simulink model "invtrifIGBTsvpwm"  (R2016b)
settings: Solver=VariableStepAuto  StartTime=0.0  StopTime=5  RelTol=1e-3
libraries: powerlib x17, powerlib_meascontrol x4

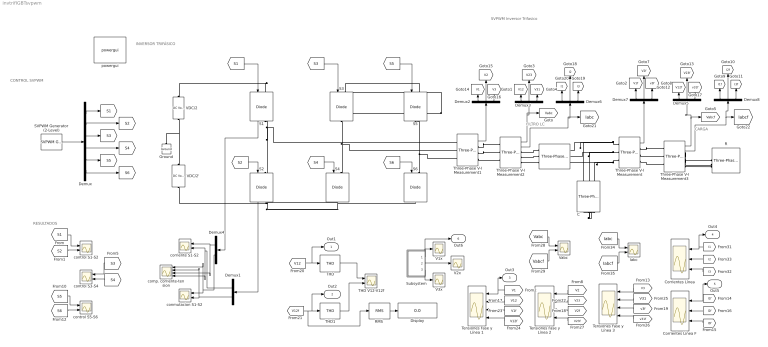
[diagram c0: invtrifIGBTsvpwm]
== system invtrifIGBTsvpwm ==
  note: RESULTADOS
  note: CONTROL SVPWM
  note: INVERSOR TRIFÁSICO
  note: SVPWM Inversor Trifasico
  note: CARGA
  note: FILTRO LC
  "C  " : powerlib/Elements/Three-Phase Series RLC Branch  LConnTagsString=A|B|C  RConnTagsString=A|B|C  BranchType=C  Resistance=1  Inductance=1e-3  Capacitance=1e-4  Measurements=None
  Corrientes Línea : Scope  NumInputPorts=3
  Corrientes Línea F : Scope  NumInputPorts=3
  Demux : Demux  Outputs=6
  Demux1 : Demux  Outputs=2
  Demux{2..3,5..8} (6 alike) : Demux  Outputs=3
  Demux4 : Demux  Outputs=2
  Display : Display
  Ground : powerlib/Elements/Ground  LConnTagsString=a
  Iabc : Scope  NumInputPorts=2
  L : powerlib/Elements/Three-Phase Series RLC Branch  LConnTagsString=A|B|C  RConnTagsString=A|B|C  BranchType=L  Resistance=40  Inductance=10e-3  Capacitance=1e-6  Measurements=Branch voltages and currents
  R : powerlib/Elements/Three-Phase Series RLC Load  LConnTagsString=A|B|C  Configuration=Y (grounded)  NominalVoltage=220  Vabc=[1e3 1e3 1e3]  Vabcp=[1e3 1e3 1e3]  NominalFrequency=50  UnbalancedPower=off  ActivePower=2430  InductivePower=1177  CapacitivePower=0  Pabc=[10e3 9e3 11e3]  QLabc=[100 90 110]  QCabc=[100 90 110]  Pabcp=[10e3 9e3 11e3]  QLabcp=[100 90 110]  QCabcp=[100 90 110]  Measurements=None  LoadType=constant Z
  "RMS " : powerlib_meascontrol/Measurements/RMS  TrueRMS=on  Freq=60  RMSInit=220  Ts=0
  S1 : powerlib/Power Electronics/IGBT//Diode  Ron=1e-3  Rs=1e5  Cs=inf  Measurements=on
  S2 : powerlib/Power Electronics/IGBT//Diode  Ron=1e-3  Rs=1e5  Cs=inf  Measurements=on
  S{3..6} (4 alike) : powerlib/Power Electronics/IGBT//Diode  Ron=1e-3  Rs=1e5  Cs=inf  Measurements=off
  SVPWM Generator (2-Level) : powerlib_meascontrol/Pulse & Signal Generators/SVPWM Generator (2-Level)  InputType=Internally generated  SwitchingPattern=Pattern #1  Fc=1050  ParUref=[0.85 -14 50]  Ts=0
  Subsystem : Subsystem
  THD : powerlib_meascontrol/Measurements/THD  Freq=60  Ts=0
  THD V12-V12f : Scope  NumInputPorts=2
  THD1 : powerlib_meascontrol/Measurements/THD  Freq=60  Ts=0
  Tensiones Fase y Línea 1 : Scope  NumInputPorts=4
  Tensiones Fase y Línea 2 : Scope  NumInputPorts=4
  Tensiones Fase y Línea 3 : Scope  NumInputPorts=4
  Three-Phase V-I Measurement : powerlib/Measurements/Three-Phase V-I Measurement  VoltageMeasurement=phase-to-ground  SetLabelV=off  LabelV=Vabc  Vpu=off  VpuLL=off  CurrentMeasurement=no  SetLabelI=off  LabelI=Iabc  Ipu=off  Pbase=100e6  Vbase=500e3  OutputType=Complex  PhasorSimulation=off  PSBequivalent=0
  Three-Phase V-I Measurement1 : powerlib/Measurements/Three-Phase V-I Measurement  VoltageMeasurement=phase-to-ground  SetLabelV=off  LabelV=Vabc  Vpu=off  VpuLL=off  CurrentMeasurement=no  SetLabelI=off  LabelI=Iabc  Ipu=off  Pbase=100e6  Vbase=500e3  OutputType=Complex  PhasorSimulation=off  PSBequivalent=0
  Three-Phase V-I Measurement2 : powerlib/Measurements/Three-Phase V-I Measurement  VoltageMeasurement=phase-to-phase  SetLabelV=off  LabelV=Vabc  Vpu=off  VpuLL=off  CurrentMeasurement=yes  SetLabelI=off  LabelI=Iabc  Ipu=off  Pbase=100e6  Vbase=500e3  OutputType=Complex  PhasorSimulation=off  PSBequivalent=0
  Three-Phase V-I Measurement3 : powerlib/Measurements/Three-Phase V-I Measurement  VoltageMeasurement=phase-to-phase  SetLabelV=off  LabelV=Vabc  Vpu=off  VpuLL=off  CurrentMeasurement=yes  SetLabelI=off  LabelI=Iabc  Ipu=off  Pbase=100e6  Vbase=500e3  OutputType=Complex  PhasorSimulation=off  PSBequivalent=0
  V1x : Scope
  V2x : Scope
  V3x : Scope
  VDC/2 : powerlib/Electrical Sources/DC Voltage Source  Amplitude=185  Measurements=None
  VDC/2' : powerlib/Electrical Sources/DC Voltage Source  Amplitude=185  Measurements=None
  "Vabc " : Scope  NumInputPorts=2
  comp. corriente-tension : Scope  NumInputPorts=4
  conmutacion S1-S2 : Scope  NumInputPorts=2
  control S1-S2 : Scope  NumInputPorts=2
  control S3-S4 : Scope  NumInputPorts=2
  "control S5-S6 " : Scope  NumInputPorts=2
  corriente S1-S2 : Scope  NumInputPorts=2
  powergui : powerlib/powergui  Priority=1  SimulationMode=Continuous  SolverType=Tustin/Backward Euler (TBE)  SampleTime=5e-5  frequency=60  SPID=off  DisableSnubberDevices=off  DisableRonSwitches=off  DisableVfSwitches=off  SwTol=0  DisplayEquations=off  Interpol=off  ExternalGateDelay=off  methode=off  Ts=10  FunctionMessages=off  echomessages=off  HookPort=off  EnableUseOfTLC=off  x0status=blocks  frequencyindice=0  Pbase=100e6  ErrMax=1e-4  Iterations=50  UnitsV=kV  UnitsW=MW  buscounter=0  RestoreLinks=warning  ResistiveCurrentMeasurement=off  Frange=[0:2:500]  Ylog=off  Xlog=on  ShowGrid=off  save=off  variable=ZData  structure=yout  ZoomFFT=off  StartTime=0.055  cycles=1  DisplayStyle=4  fundamental=50  FreqAxis=off  MaxFrequency=7800  frequencyindicesteady=1  RmsSteady=1  display=off
  Out1 : Outport  SignalName=V12
  Out2 : Outport  Port=2  SignalName=V12f
  Out3 : Outport  Port=3  SignalName=V1
  Out4 : Outport  Port=4  SignalName=I1
  Out5 : Outport  Port=5  SignalName=I1f
  Out6 : Outport  Port=6  SignalName=V1x
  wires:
  SVPWM Generator (2-Level)/1 -> Demux/1
  [S1] -> S1/1
  [S2] -> S2/1
  [S3] -> S3/1
  [S4] -> S4/1
  [S6] -> S6/1
  [S5] -> S5/1
  Demux/2 -> [S2]
  Demux/1 -> [S1]
  Demux/3 -> [S3]
  Demux/4 -> [S4]
  Demux/5 -> [S5]
  Demux/6 -> [S6]
  [S1] -> control S1-S2/1
  [S2] -> control S1-S2/2
  [S3] -> control S3-S4/1
  [S4] -> control S3-S4/2
  [S5] -> "control S5-S6 "/1
  [S6] -> "control S5-S6 "/2
  S2/1 -> Demux1/1
  S1/1 -> Demux4/1
  Demux1/1 -> comp. corriente-tension/4, corriente S1-S2/2
  Demux4/1 -> comp. corriente-tension/3, corriente S1-S2/1
  Demux4/2 -> comp. corriente-tension/1, conmutacion S1-S2/1
  Demux1/2 -> comp. corriente-tension/2, conmutacion S1-S2/2
  Three-Phase V-I Measurement/1 -> Demux7/1
  Demux7/1 -> [V1f]
  Demux7/2 -> [V2f]
  Demux7/3 -> [v3f]
  Demux8/2 -> [I2f]
  Demux8/1 -> [I1f]
  Demux8/3 -> [I3f]
  Three-Phase V-I Measurement1/1 -> Demux2/1
  Demux2/2 -> [V2]
  Demux2/3 -> [V3]
  Three-Phase V-I Measurement2/1 -> Demux3/1, [Vabc]
  Demux3/1 -> [V12]
  Demux3/2 -> [V23]
  Demux3/3 -> [V31]
  Three-Phase V-I Measurement3/1 -> Demux5/1, [Vabcf]
  Demux5/1 -> [V12f]
  Demux5/2 -> [V23f]
  Demux5/3 -> [v31f]
  Three-Phase V-I Measurement3/2 -> Demux8/1, [Iabcf]
  Demux2/1 -> [V1]
  Three-Phase V-I Measurement2/2 -> [Iabc], Demux6/1
  Demux6/2 -> [I2]
  Demux6/1 -> [I1]
  Demux6/3 -> [I3]
  [V1] -> Out3/1, Tensiones Fase y Línea 1/1
  [V2] -> Tensiones Fase y Línea 2/1
  [V2f] -> Tensiones Fase y Línea 2/3
  [V23] -> Tensiones Fase y Línea 2/2
  [I2f] -> Corrientes Línea F/2
  [I1f] -> Out5/1, Corrientes Línea F/1
  [I3f] -> Corrientes Línea F/3
  [V12] -> Tensiones Fase y Línea 1/2
  [V3] -> Tensiones Fase y Línea 3/1
  [v3f] -> Tensiones Fase y Línea 3/3
  [V1f] -> Tensiones Fase y Línea 1/3
  [V12f] -> Tensiones Fase y Línea 1/4
  [V31] -> Tensiones Fase y Línea 3/2
  [v31f] -> Tensiones Fase y Línea 3/4
  [V23f] -> Tensiones Fase y Línea 2/4
  THD/1 -> THD V12-V12f/1
  [V12] -> Out1/1, THD/1
  THD1/1 -> THD V12-V12f/2
  [Vabc] -> "Vabc "/1
  [Vabcf] -> "Vabc "/2
  [V12f] -> "RMS "/1, Out2/1, THD1/1
  "RMS "/1 -> Display/1
  [I2] -> Corrientes Línea/2
  [I1] -> Out4/1, Corrientes Línea/1
  [I3] -> Corrientes Línea/3
  [Iabc] -> Iabc/1
  [Iabcf] -> Iabc/2
  Subsystem/2(Out2) -> V2x/1
  Subsystem/3(Out3) -> V3x/1
  Subsystem/1(Out1) -> Out6/1, V1x/1
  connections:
  VDC/2'/LConn1 -- S2/RConn1 -- S6/RConn1 -- S4/RConn1
  VDC/2/RConn1 -- S1/LConn1 -- S5/LConn1 -- S3/LConn1
  S5/RConn1 -- Three-Phase V-I Measurement1/LConn3 -- S6/LConn1
  VDC/2/LConn1 -- Ground/LConn1 -- VDC/2'/RConn1
  S3/RConn1 -- Three-Phase V-I Measurement1/LConn2 -- S4/LConn1
  S1/RConn1 -- Three-Phase V-I Measurement1/LConn1 -- S2/LConn1
  Three-Phase V-I Measurement/LConn1 -- L/RConn1 -- "C  "/LConn1
  Three-Phase V-I Measurement/LConn2 -- L/RConn2 -- "C  "/LConn2
  Three-Phase V-I Measurement/LConn3 -- L/RConn3 -- "C  "/LConn3
  "C  "/RConn2 -- "C  "/RConn1 -- "C  "/RConn3
  Three-Phase V-I Measurement/RConn2 -- Three-Phase V-I Measurement3/LConn2
  Three-Phase V-I Measurement3/RConn1 -- R/LConn1
  L/LConn1 -- Three-Phase V-I Measurement2/RConn1
  Three-Phase V-I Measurement1/RConn2 -- Three-Phase V-I Measurement2/LConn2
  Three-Phase V-I Measurement3/RConn2 -- R/LConn2
  Three-Phase V-I Measurement1/RConn1 -- Three-Phase V-I Measurement2/LConn1
  Three-Phase V-I Measurement/RConn1 -- Three-Phase V-I Measurement3/LConn1
  L/LConn2 -- Three-Phase V-I Measurement2/RConn2
  Three-Phase V-I Measurement1/RConn3 -- Three-Phase V-I Measurement2/LConn3
  Three-Phase V-I Measurement3/RConn3 -- R/LConn3
  L/LConn3 -- Three-Phase V-I Measurement2/RConn3
  Three-Phase V-I Measurement/RConn3 -- Three-Phase V-I Measurement3/LConn3

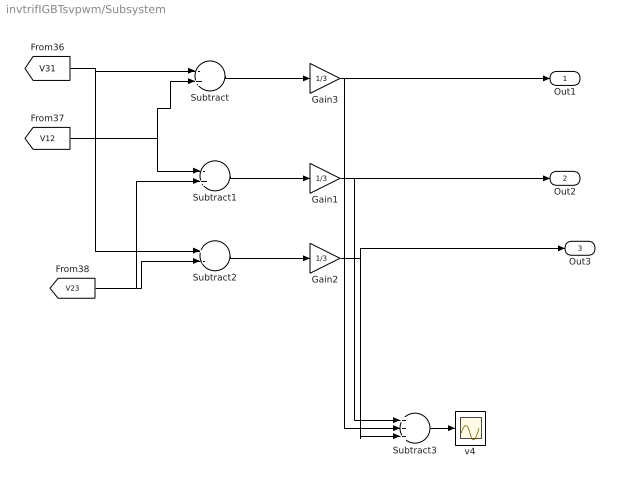
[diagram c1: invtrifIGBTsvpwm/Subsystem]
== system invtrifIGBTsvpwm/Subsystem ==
  Gain1 : Gain  Gain=1/3
  Gain2 : Gain  Gain=1/3
  Gain3 : Gain  Gain=1/3
  Subtract : Sum  Inputs=-+
  Subtract1 : Sum  Inputs=-+
  Subtract2 : Sum  Inputs=+-
  Subtract3 : Sum  Inputs=+++
  v4 : Scope
  Out1 : Outport
  Out2 : Outport  Port=2
  Out3 : Outport  Port=3
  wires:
  [V23] -> Subtract1/2, Subtract2/2
  Subtract3/1 -> v4/1
  [V12] -> Subtract/2, Subtract1/1
  [V31] -> Subtract2/1, Subtract/1
  Subtract2/1 -> Gain2/1
  Subtract1/1 -> Gain1/1
  Gain2/1 -> Out3/1, Subtract3/3
  Gain1/1 -> Out2/1, Subtract3/1
  Gain3/1 -> Out1/1, Subtract3/2
  Subtract/1 -> Gain3/1
